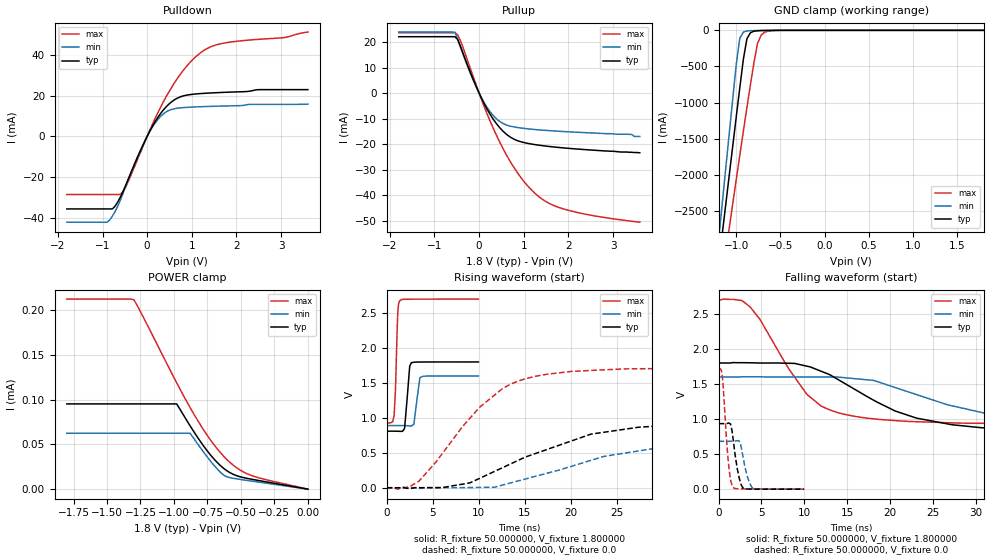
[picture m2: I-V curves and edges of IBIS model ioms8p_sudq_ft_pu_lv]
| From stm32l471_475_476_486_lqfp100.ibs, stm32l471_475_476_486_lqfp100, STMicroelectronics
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|   Model ioms8p_sudq_ft_pu_lv
[Model]  ioms8p_sudq_ft_pu_lv
Model_type I/O
Polarity   Non-Inverting
Enable   Active-Low
Vinl =   0.540000V
Vinh =   1.260000V
Vmeas =  0.900000V
Cref =   50.000000pF
Rref =   100.000000M
Vref =   0.0V
C_comp   1.984800pF   1.899400pF   2.077500pF
[Temperature Range]   25.000000   -40.000000   0.125000k
[Pullup Reference]   1.800000V   1.600000V   2.700000V
[Pulldown Reference]   0.0V   0.0V   0.0V
[POWER Clamp Reference]   1.800000V   1.600000V   2.700000V
[GND Clamp Reference]   0.0V   0.0V   0.0V
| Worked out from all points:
|   slope of the pulldown table from 0 to 0.27 V, typ, clamps not added: 26.4 ohm
|   slope of the pullup table from 0 to 0.27 V, typ, clamps not added: 30.1 ohm
|   GND clamp passes 1 mA (typ) near -0.61 V on its own axis
|   rising waveform, R_fixture 50.000000, V_fixture 1.800000: 20-80 % time 371ps typ, 419ps min, 254ps max; typ from 0.81 V to 1.8 V
|   rising waveform, R_fixture 50.000000, V_fixture 0.0: 20-80 % time 10.8ns typ, 12.9ns min, 6.96ns max; typ from 0.001 V to 0.935 V
|   falling waveform, R_fixture 50.000000, V_fixture 1.800000: 20-80 % time 9.93ns typ, 12.5ns min, 5.81ns max; typ from 1.8 V to 0.81 V
|   falling waveform, R_fixture 50.000000, V_fixture 0.0: 20-80 % time 694ps typ, 759ps min, 590ps max; typ from 0.935 V to 0.001 V
[Pulldown]
|Voltage   I(typ)   I(min)   I(max)
-1.8V     -35.64mA   -42.15mA   -28.59mA
-900mV    -35.64mA   -42.15mA   -28.59mA
-780mV    -35.64mA   -39.2mA    -28.59mA
-600mV    -29.83mA   -31.3mA    -28.52mA
-420mV    -20.8mA    -21.07mA   -21.98mA
60mV      2.604mA    2.459mA    3.062mA
240mV     9.303mA    8.31mA     11.61mA
480mV     15.67mA    12.64mA    21.52mA
720mV     19.18mA    13.9mA     29.74mA
960mV     20.46mA    14.3mA     36.27mA
1.44V     21.29mA    14.7mA     44.06mA
3.6V      22.91mA    15.79mA    51.15mA
[Pullup]
|Voltage   I(typ)   I(min)   I(max)
-1.8V     22.09mA    23.9mA     23.64mA
-540mV    22.09mA    23.85mA    23.64mA
-480mV    21.02mA    21.11mA    22.74mA
-60mV     2.392mA    2.26mA     2.893mA
300mV     -9.801mA   -8.48mA    -13.12mA
480mV     -13.91mA   -11.33mA   -19.82mA
720mV     -17.48mA   -13.04mA   -27.45mA
1.02V     -19.45mA   -13.87mA   -34.96mA
1.32V     -20.37mA   -14.39mA   -40.32mA
1.62V     -21.02mA   -14.78mA   -43.66mA
2.04V     -21.71mA   -15.22mA   -46.12mA
3.6V      -23.4mA    -17mA      -50.6mA
[GND_clamp]
|Voltage   I(typ)   I(min)   I(max)
-1.8V     -9.477A    -9.805A    -9.016A
-1.2V     -3.243A    -2.9A      -3.759A
-1.16V    -2.83A     -2.409A    -3.417A
-1.12V    -2.418A    -1.919A    -3.076A
-1.08V    -2.008A    -1.431A    -2.736A
-1V       -1.194A    -466mA     -2.061A
-960mV    -792.8mA   -108.7mA   -1.727A
-920mV    -402mA     -24.35mA   -1.396A
-880mV    -117.8mA   -9.188mA   -1.071A
-760mV    -5.896mA   -2.88mA    -183.8mA
-680mV    -2.395mA   -1.099mA   -26.61mA
1.8V      0A         0A         0A
[POWER_clamp]
|Voltage   I(typ)   I(min)   I(max)
-1.8V     95.27uA    62.52uA    212.4uA
-1.3V     95.27uA    62.52uA    211.7uA
-1.24V    95.27uA    62.52uA    195.4uA
-980mV    95.27uA    62.52uA    119uA
-880mV    70.93uA    62.52uA    91.35uA
-740mV    40.61uA    33.79uA    57.65uA
-640mV    24.64uA    16.99uA    38.63uA
-600mV    20.11uA    13.6uA     32.43uA
-540mV    15.51uA    11.72uA    24.8uA
-440mV    11.66uA    9.491uA    16.35uA
-340mV    8.934uA    7.326uA    11.65uA
0V        0A         0A         0A
[Ramp]
| variable   typ   min   max
dV/dt_r  0.55941/10.79580n   0.40761/12.82955n   1.02729/6.95129n
dV/dt_f  0.58889/9.90915n   0.41170/12.44957n   1.06297/5.80742n
R_load = 50.000000
[Rising Waveform]
R_fixture= 50.000000
V_fixture= 1.800000
V_fixture_min= 1.600000
V_fixture_max= 2.700000
|time   V(typ)   V(min)   V(max)
0s        809.8mV    890.3mV    928mV
800.8ps   809.8mV    890.3mV    1.024V
961ps     809.7mV    890.3mV    1.426V
1.201ns   809.4mV    890.3mV    2.493V
1.461ns   807.3mV    890.3mV    2.681V
1.942ns   848.8mV    889.7mV    2.697V
2.503ns   1.739V     885mV      2.698V
2.683ns   1.79V      882.7mV    2.698V
3.624ns   1.799V     1.579V     2.698V
9.97ns    1.8V       1.6V       2.7V
[Rising Waveform]
R_fixture= 50.000000
V_fixture= 0.0
V_fixture_min= 0.0
V_fixture_max= 0.0
|time   V(typ)   V(min)   V(max)
0s        728.2uV    547.5uV    1.27mV
1.201ns   748.8uV    546.1uV    -19.75mV
3.504ns   2.314mV    -7.576mV   93.88mV
10.11ns   135.3mV    5.523mV    1.152V
12.71ns   295mV      43.05mV    1.429V
15.32ns   450.8mV    133.8mV    1.568V
22.22ns   767.9mV    393mV      1.679V
27.33ns   865.1mV    526mV      1.703V
31.53ns   900.8mV    613mV      1.708V
49.85ns   935.3mV    683.1mV    1.715V
[Falling Waveform]
R_fixture= 50.000000
V_fixture= 1.800000
V_fixture_min= 1.600000
V_fixture_max= 2.700000
|time   V(typ)   V(min)   V(max)
0s        1.8V       1.6V       2.7V
2.703ns   1.805V     1.604V     2.691V
3.604ns   1.803V     1.603V     2.607V
10.31ns   1.754V     1.6V       1.351V
12.01ns   1.679V     1.6V       1.182V
13.91ns   1.565V     1.599V     1.091V
20.62ns   1.114V     1.449V     978.6mV
27.13ns   921.4mV    1.192V     946.4mV
34.23ns   850.4mV    995.9mV    935.6mV
49.85ns   809.8mV    890.3mV    928mV
[Falling Waveform]
R_fixture= 50.000000
V_fixture= 0.0
V_fixture_min= 0.0
V_fixture_max= 0.0
|time   V(typ)   V(min)   V(max)
0s        935.3mV    683.1mV    1.715V
440.4ps   935.2mV    683.1mV    1.599V
1.121ns   942.3mV    683mV      404.6mV
1.381ns   931.5mV    682.9mV    148.2mV
1.662ns   743.6mV    682.4mV    31.23mV
2.362ns   180.6mV    692.5mV    5.887mV
2.823ns   20.98mV    478.4mV    5.182mV
3.584ns   2.007mV    96.88mV    4.863mV
4.164ns   1.186mV    4.284mV    4.257mV
9.97ns    728.2uV    547.5uV    1.27mV
